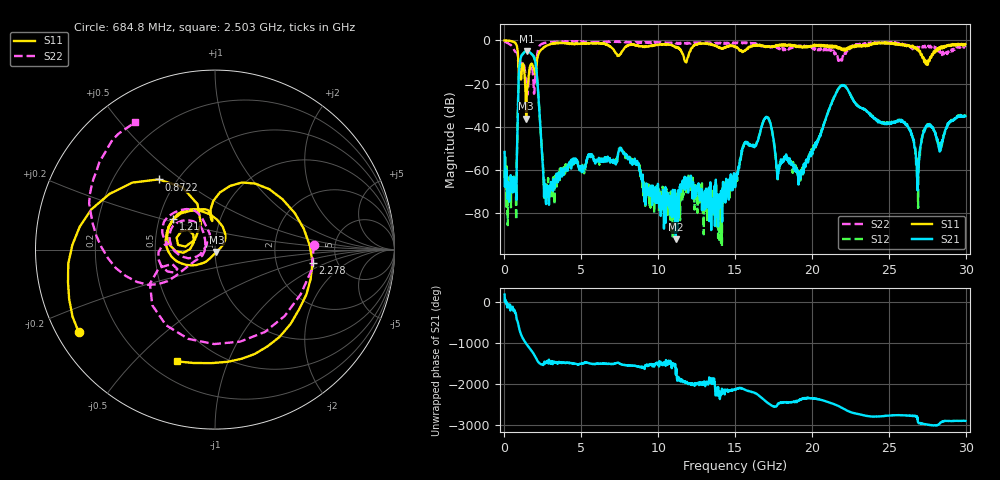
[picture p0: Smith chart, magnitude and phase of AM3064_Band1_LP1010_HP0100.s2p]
# Hz S DB R 50.0
!freq dBS11 angS11 dBS21 angS21 dBS12 angS12 dBS22 angS22
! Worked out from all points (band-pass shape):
!   1600 points, 10 MHz to 29.98 GHz, reference 50 ohm
!   highest |S21| = -4.87 dB at 1.453 GHz (marker M1); lowest = -92.1 dB at 11.14 GHz (marker M2)
!   |S21| within 3 dB of the highest: 1.068 GHz to 1.927 GHz (858.9 MHz wide, 57.3 % of centre)
!   lowest |S11| = -36.3 dB at 1.416 GHz (marker M3), VSWR 1.03, Z = 50.8 - j1.31 ohm
!   |S11| at or under -10 dB: 902 MHz to 2.108 GHz (1.206 GHz wide, 80.1 % of centre); 27.39303 GHz to 27.45806 GHz (65.03 MHz wide, 0.237 % of centre); 27.48879 GHz to 27.56295 GHz (74.17 MHz wide, 0.269 % of centre)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
!   |S22| runs from -25.1 to -0.4 dB; largest |S21 - S12| = 0.008
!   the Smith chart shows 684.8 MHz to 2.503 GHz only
!   S11 on the Smith chart (normalised r, x): 684.8 MHz: 0.06, -0.28; 872.2 MHz: 0.40, +0.42; 1.21 GHz: 0.59, +0.22; 2.278 GHz: 3.27, -0.68; 2.503 GHz: 0.31, -0.67
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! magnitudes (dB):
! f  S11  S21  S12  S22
! 10 MHz  0.0  -51.7  -63.8  -0.4
! 684.8 MHz  -1.0  -65.7  -65.4  -5.2
! 872.2 MHz  -6.0  -30.9  -30.8  -7.8
! 1.21 GHz  -10.8  -6.2  -6.1  -9.9
! 1.416 GHz  -36.3  -4.9  -4.9  -20.4
! 1.453 GHz  -24.7  -4.9  -4.9  -22.0
! 1.959 GHz  -14.4  -8.6  -8.5  -22.4
! 2.278 GHz  -5.2  -33.4  -33.3  -2.5
! 2.503 GHz  -3.6  -58.4  -57.5  -1.5
! 5.015 GHz  -1.4  -58.8  -59.0  -0.7
! 7.601 GHz  -5.8  -51.0  -50.0  -0.7
! 10 GHz  -2.0  -69.4  -69.6  -0.9
! 11.14 GHz  -3.4  -92.1  -78.1  -1.4
! 15 GHz  -3.0  -68.1  -63.1  -1.4
! 17.03 GHz  -3.0  -35.4  -35.4  -3.1
! 17.8 GHz  -2.1  -61.5  -60.6  -3.4
! 19.99 GHz  -2.8  -51.4  -51.4  -3.3
! 21.94 GHz  -4.2  -20.9  -21.0  -9.4
! 25 GHz  -1.0  -38.3  -38.1  -1.0
! 26.89 GHz  -4.1  -64.0  -70.7  -3.5
! 27.49 GHz  -10.0  -39.5  -39.2  -3.0
! 29.98 GHz  -1.7  -35.1  -35.4  -3.1
